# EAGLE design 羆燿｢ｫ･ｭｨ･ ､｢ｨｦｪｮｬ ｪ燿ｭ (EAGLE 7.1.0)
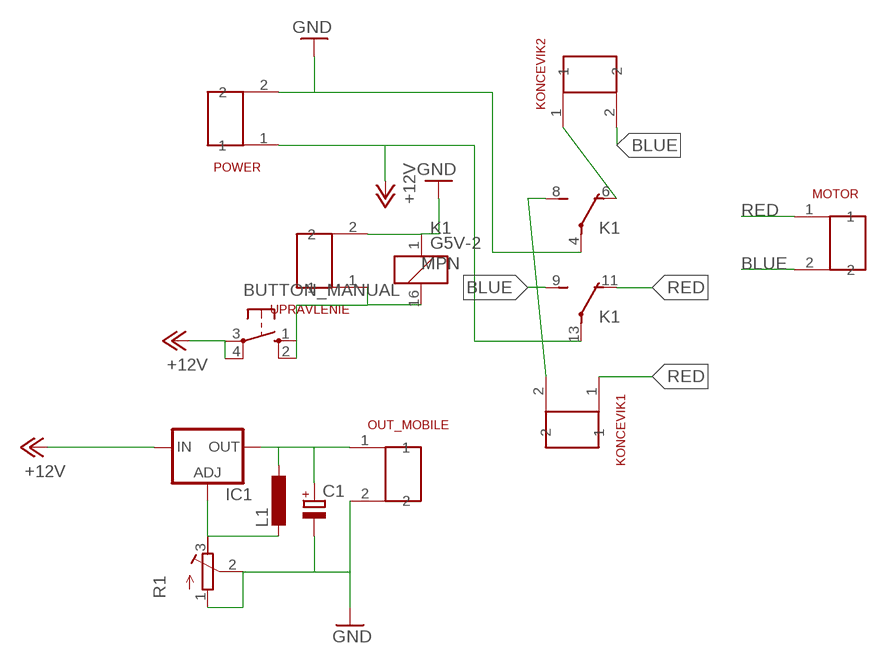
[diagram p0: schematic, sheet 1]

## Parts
BUTTON_MANUAL  10-XX  [B3F-10XX]
C1  CPOL-EUE2.5-7  [E2,5-7]
IC1  LM317TS  [317TS]
K1  G5V-2  [G5V-2]
KONCEVIK1  CON2X2.54  [CON2X2.54]
KONCEVIK2  CON2X2.54  [CON2X2.54]
L1  L-EU0207/7  [0207/7]
MOTOR  CON2X2.54  [CON2X2.54]
OUT_MOBILE  CON2X2.54  [CON2X2.54]
POWER  CON2X2.54  [CON2X2.54]
R1  R-TRIMM3339P  [RTRIM3339P]
UPRAVLENIE  CON2X2.54  [CON2X2.54]

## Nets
+12V: BUTTON_MANUAL.3(P) BUTTON_MANUAL.4(P1) IC1.3(IN) K1.13(2:P) POWER.1
BLUE: K1.9(2:S) KONCEVIK2.2 MOTOR.2
GND: C1.- K1.1 K1.4(1:P) OUT_MOBILE.2 POWER.2 R1.1(E) R1.2(S) UPRAVLENIE.2
N$2: BUTTON_MANUAL.1(S) BUTTON_MANUAL.2(S1) K1.16 UPRAVLENIE.1
N$3: C1.+ IC1.2(OUT) L1.1 OUT_MOBILE.1
N$5: K1.6(1:O) KONCEVIK2.1
N$6: IC1.1(ADJ) L1.2 R1.3(A)
N$7: K1.8(1:S) KONCEVIK1.2
RED: K1.11(2:O) KONCEVIK1.1 MOTOR.1

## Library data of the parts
BUTTON_MANUAL = switch-omron:10-XX: OMRON SWITCH; MPN: B3F-1000; OC_FARNELL: 176432; OC_NEWARK: 36M3542
C1 = resistor:CPOL-EU: POLARIZED CAPACITOR, European symbol
IC1 = v-reg:LM317TS: VOLTAGE REGULATOR
K1 = relay:G5V-2: OMRON PCB Relay Source: http://www.omron.com/ecb/products/pdf/en-g5v2.pdf; MPN: G5V-2 5DC; OC_FARNELL: 9949488; OC_NEWARK: 78K5703
KONCEVIK1 KONCEVIK2 MOTOR OUT_MOBILE POWER UPRAVLENIE = my:CON2X2.54
L1 = resistor:L-EU: INDUCTOR, European symbol
R1 = resistor:R-TRIMM: Trimm resistor

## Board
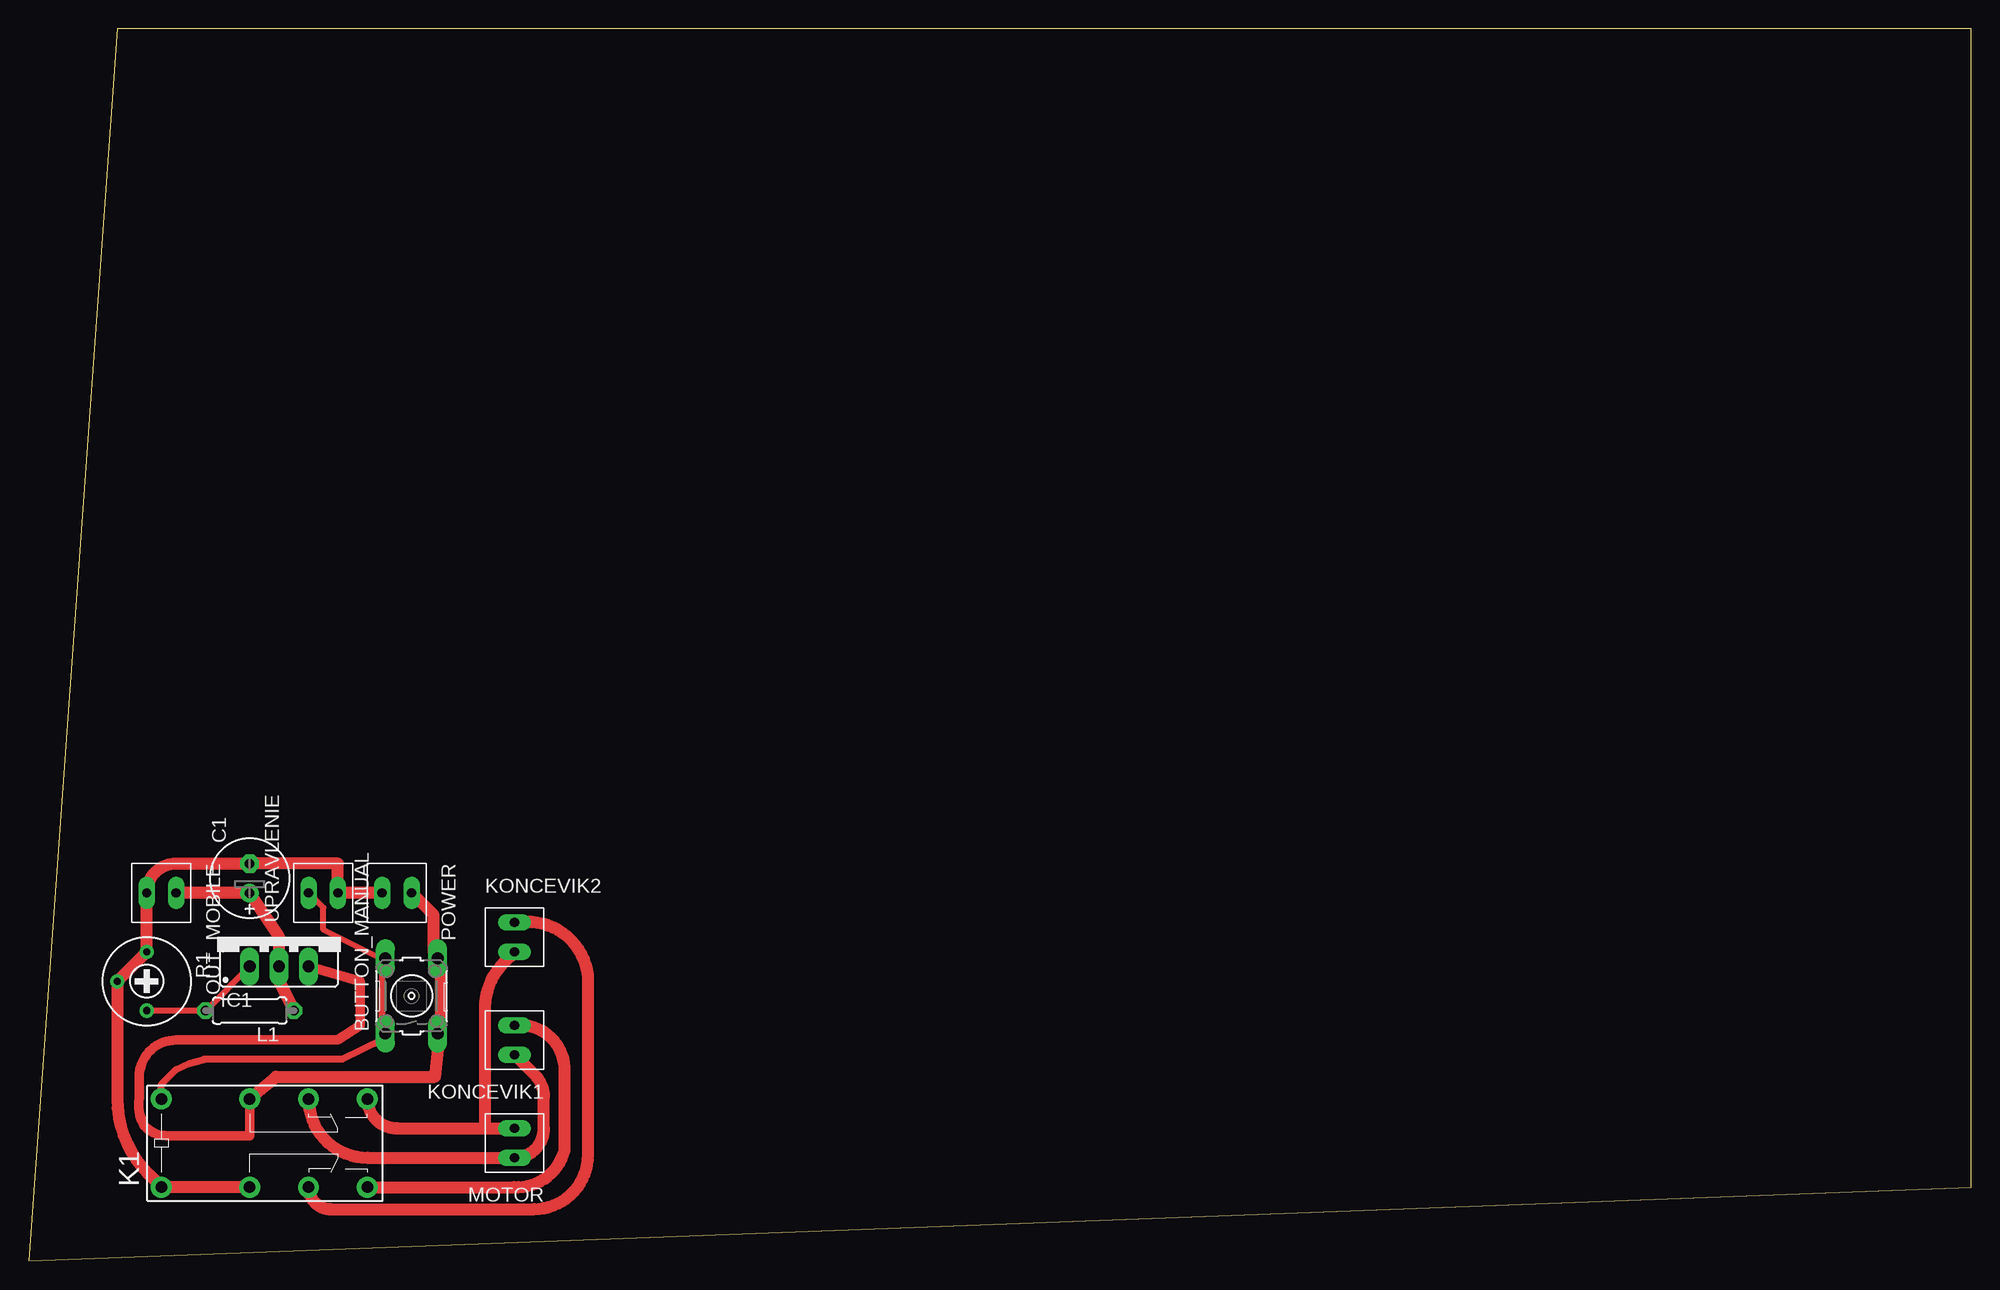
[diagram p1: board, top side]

Size 167.62 x 106.35 mm. Coordinates in mm from the lower left corner, seen from the top.
Outline: 0,0 167.62,6.35 167.62,106.35 7.62,106.35 0,0
Copper layers (1*16): Top 0.035mm / dielectric 1.5mm / Bottom 0.035mm
Design rules "default": minimum track width 20mil, minimum drill 32mil, track to track 14mil, track to pad 14mil, pad to pad 14mil, via to via 14mil, smd to smd 8mil, copper to edge 40mil, drill to drill 40mil, minimum pad ring 12mil, minimum via ring 12mil, stop-mask expansion 4mil, vias tented up to drill 0mil, thermal gap 10mil

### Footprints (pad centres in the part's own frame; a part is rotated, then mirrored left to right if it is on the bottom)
B3F-10XX = drill 1.016 long: 1 -3.251,2.261; 2 3.251,2.261; 3 -3.251,-2.261; 4 3.251,-2.261
E2,5-7 = drill 0.813 pad 1.6: + -1.27,0 | drill 0.813 pad 1.6 octagon: - 1.27,0
317TS = drill 1.016 long: 1 -2.54,-2.54; 2 0,-2.54; 3 2.54,-2.54
G5V-2 = drill 1 pad 1.8: 1 -8.89,-3.81; 4 -1.27,-3.81; 6 3.81,-3.81; 8 8.89,-3.81; 9 8.89,3.81; 11 3.81,3.81; 13 -1.27,3.81; 16 -8.89,3.81
CON2X2.54 = drill 0.8 long: 1 0,1.27; 2 0,-1.27
0207/7 = drill 0.813 octagon: 1 -3.81,0; 2 3.81,0
RTRIM3339P = drill 0.61: 1 -2.54,0; 2 0,-2.54; 3 2.54,0

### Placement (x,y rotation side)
BUTTON_MANUAL  33.02,22.86 90 top
C1  19.05,33.02 90 top
IC1  21.59,27.94 0 top
K1  20.32,10.16 0 top
KONCEVIK1  41.91,19.05 180 top
KONCEVIK2  41.91,27.94 0 top
L1  19.05,21.59 180 top
MOTOR  41.91,10.16 180 top
OUT_MOBILE  11.43,31.75 270 top
POWER  31.75,31.75 270 top
R1  10.16,24.13 270 top
UPRAVLENIE  25.4,31.75 90 top

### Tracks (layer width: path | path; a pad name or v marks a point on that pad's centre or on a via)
+12V
  Top 0.508: 34.92,26.67 BUTTON_MANUAL.4 35.56,26.03 | 35.56,19.69 BUTTON_MANUAL.3 35.43,19.05
  Top 0.813: IC1.3 28.57,24.13 28.57,20.32 26.67,19.05 12.7,19.05 arc90 9.53,15.88 9.53,14.02 arc45 10.01,11.58 arc45 11.91,10.79 19.05,10.79 K1.13
  Top 1.016: POWER.1 34.92,29.84 34.92,26.67 | 35.56,26.03 35.56,19.69 | 35.43,19.05 35.05,15.88 21.34,15.88 K1.13
BLUE
  Top 1.016: K1.9 arc90 31.75,11.43 39.37,11.43 | 39.37,11.43 MOTOR.2 | 39.37,11.43 39.37,21.78 arc-45 41.03,25.79 KONCEVIK2.2
GND
  Top 1.016: POWER.2 UPRAVLENIE.2 26.67,34.29 C1.- 12.7,34.29 arc90 OUT_MOBILE.2 R1.1 R1.2 7.62,13.99 arc45 10.33,7.45 K1.1 K1.4
N$2
  Top 0.508: UPRAVLENIE.1 25.4,30.48 25.4,28.58 30.48,26.03 | 30.48,23.49 30.48,26.03 | 30.48,26.03 BUTTON_MANUAL.2
  Top 0.61: 30.48,23.49 30.48,19.69 BUTTON_MANUAL.1 30.48,19.05 27.05,17.4 15.11,17.4 13.84,17.02 12.7,16.51 11.43,15.24 K1.16
N$3
  Top 0.508: IC1.2 21.59,24.13
  Top 1.016: OUT_MOBILE.1 C1.+ 21.59,27.94 IC1.2 | 21.59,24.13 L1.1
N$5
  Top 1.016: KONCEVIK2.1 42.41,29.21 arc-90 48.26,24.63 48.26,9.13 arc-90 43.57,4.44 26.04,4.44 arc-90 K1.6
N$6
  Top 0.508: R1.3 L1.2 IC1.1
N$7
  Top 1.016: KONCEVIK1.2 42.13,20.32 arc-90 46.23,16.73 46.23,9.52 arc-79 41.85,6.35 K1.8
RED
  Top 1.016: K1.11 arc90 29.21,8.89 MOTOR.1 arc90 44.45,11.43 44.45,14.19 arc45 43.71,15.98 KONCEVIK1.1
